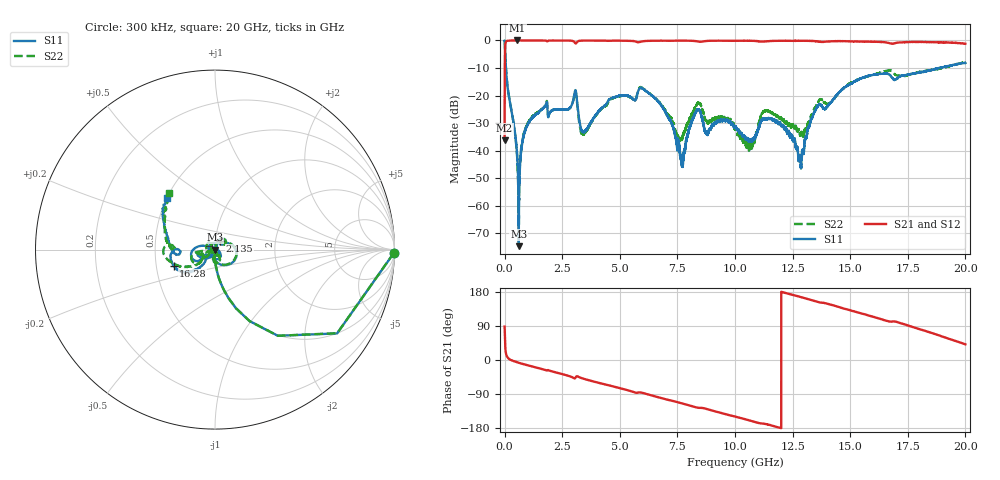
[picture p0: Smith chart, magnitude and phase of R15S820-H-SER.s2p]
!{R15S820}
!Johanson Technology Inc.
!www.johansontechnology.com
!Test Board Conditions:
!Substrate Type  RO4350B
!Substrate Thickness  20 mil
!Substrate Dk  3.66
!TL Type: GCPW
!TL Trace Width  34 mil
!TL Gap  10 mil
!Electrode orientation  Horizontal
!DUT TOPOLOGY	SERIES
!Mounting Pad LxW  26x52 mil
! Created Sat Feb  6 14:37:01 2021
# hz S ma R 50
! 2 Port Network Data from SP1.SP block
! freq  magS11  angS11  magS21  angS21  magS12  angS12  magS22  angS22
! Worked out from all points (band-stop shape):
!   20001 points, 300 kHz to 20 GHz, reference 50 ohm
!   highest |S21| = 0.00 dB at 547.3 MHz (marker M1); lowest = -36.3 dB at 300 kHz (marker M2)
!   |S21| within 3 dB of the highest: 19.57 MHz to end of sweep
!   lowest |S11| = -74.6 dB at 616.3 MHz (marker M3), VSWR 1.00, Z = 50 - j0.00956 ohm
!   |S11| at or under -10 dB: 57.86 MHz to 18.84 GHz (18.78 GHz wide, 199 % of centre); 18.84178 GHz to 18.8467 GHz (4.92 MHz wide, 0.0261 % of centre); 18.84762 GHz to 18.85398 GHz (6.354 MHz wide, 0.0337 % of centre)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
!   |S22| runs from -67.0 to 0.0 dB; largest |S21 - S12| = 0.016
!   S11 on the Smith chart (normalised r, x): 300 kHz: open; 2.135 GHz: 1.05, +0.10; 16.28 GHz: 0.62, -0.12; 20 GHz: 0.50, +0.34
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300000  0.9968 -1.1  0.01539 88.3  0.01544 88.8  0.9971 -1.0
1.103e8  0.1695 -81.6  0.9843 8.4  0.9854 8.3  0.1698 -81.5
5.473e8  0.007734 -97.6  0.9999 -6.1  0.9994 -6.1  0.007321 -95.6
6.163e8  0.0001857 -149.0  0.9996 -7.4  0.9992 -7.4  0.001003 117.2
1.0413e9  0.03188 76.5  0.9989 -14.6  0.9984 -14.6  0.03326 75.5
2.1353e9  0.05536 60.8  0.9964 -31.3  0.9964 -31.3  0.05502 56.0
3.0603e9  0.1235 -11.5  0.8989 -48.1  0.8993 -48.1  0.1213 -9.1
3.3343e9  0.02351 -107.7  0.992 -47.6  0.9914 -47.6  0.02065 -134.4
4.6893e9  0.09104 -152.3  0.9907 -69.4  0.9906 -69.4  0.08906 -163.8
6.6673e9  0.07855 164.0  0.9897 -98.2  0.9898 -98.2  0.07908 -174.1
7.6983e9  0.00669 78.8  0.9907 -114.5  0.9917 -114.4  0.01561 -97.2
8.3773e9  0.05544 -64.1  0.9604 -125.8  0.9595 -125.8  0.07275 -73.8
8.7653e9  0.02029 -75.0  0.9771 -129.1  0.9783 -129.1  0.03494 -87.2
1.00003e10  0.02752 -82.6  0.9856 -149.2  0.9864 -149.2  0.02571 -72.2
1.06713e10  0.01481 -100.5  0.9878 -160.2  0.9861 -160.2  0.01305 -96.0
1.12023e10  0.03798 162.6  0.9514 -167.7  0.9525 -167.7  0.04855 172.2
1.16353e10  0.03625 97.0  0.9811 -173.7  0.9807 -173.6  0.0476 123.8
1.28253e10  0.007531 -6.7  0.9834 166.6  0.9839 166.7  0.01948 158.8
1.33343e10  0.03887 -113.5  0.9796 157.7  0.9796 157.6  0.04478 -138.2
1.62753e10  0.2473 -158.9  0.9414 109.1  0.9372 108.9  0.259 -165.0
1.66673e10  0.2428 -175.3  0.9031 101.9  0.8894 101.9  0.2883 -175.5
2e10  0.3909 132.3  0.8706 41.4  0.8617 41.2  0.4088 128.6
